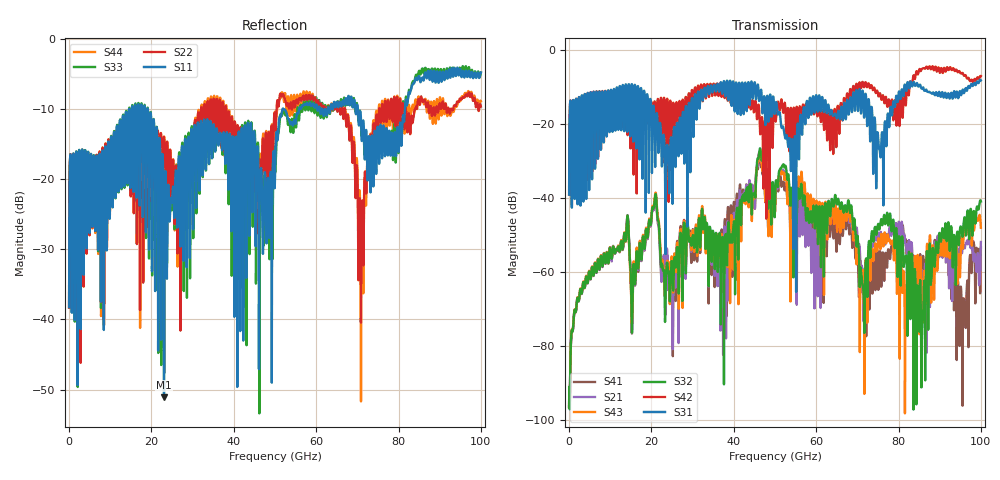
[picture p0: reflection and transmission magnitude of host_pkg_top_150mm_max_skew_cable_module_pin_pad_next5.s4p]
# Hz S RI R 50
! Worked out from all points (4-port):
!   10000 points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, 10 MHz to 100 GHz, reference 50 ohm
!   strongest paths, dB at 10 MHz, 25.01 GHz, 50.01 GHz, 75.01 GHz, 100 GHz:
!     S31: -39.0, -29.1, -15.5, -22.8, -8.1
!     S42: -39.1, -23.6, -16.0, -11.7, -6.9
!     S32: -96.3, -57.6, -41.9, -47.1, -40.9
!     S43: -96.5, -56.8, -43.6, -51.9, -48.0
!     S21: -96.4, -61.5, -40.1, -49.3, -51.8
!     S41: -96.6, -59.1, -43.1, -60.0, -53.3
!   lowest |S11| = -51.1 dB at 23.05 GHz (marker M1), VSWR 1.01, Z = 50.2 + j0.147 ohm
!   |S11| at or under -10 dB: start of sweep to 14.56 GHz; 19.08 GHz to 51.81 GHz (32.74 GHz wide, 92.4 % of centre); 70.14 GHz to 81.56 GHz (11.42 GHz wide, 15.1 % of centre)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
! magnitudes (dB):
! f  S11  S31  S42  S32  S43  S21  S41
! 10 MHz  -38.2  -39.0  -39.1  -96.3  -96.5  -96.4  -96.6
! 20.75 GHz  -16.5  -19.7  -13.8  -41.0  -40.5  -41.5  -41.1
! 23.05 GHz  -51.1  -23.5  -12.8  -59.9  -60.0  -55.5  -58.3
! 46.46 GHz  -19.2  -11.3  -22.4  -26.7  -28.1  -28.7  -30.3
! 54.78 GHz  -11.6  -23.6  -20.2  -38.5  -37.9  -42.9  -41.1
! 85.4 GHz  -6.1  -9.9  -5.6  -68.8  -57.2  -73.1  -59.6
! 100 GHz  -4.7  -8.1  -6.9  -40.9  -48.0  -51.8  -53.3
